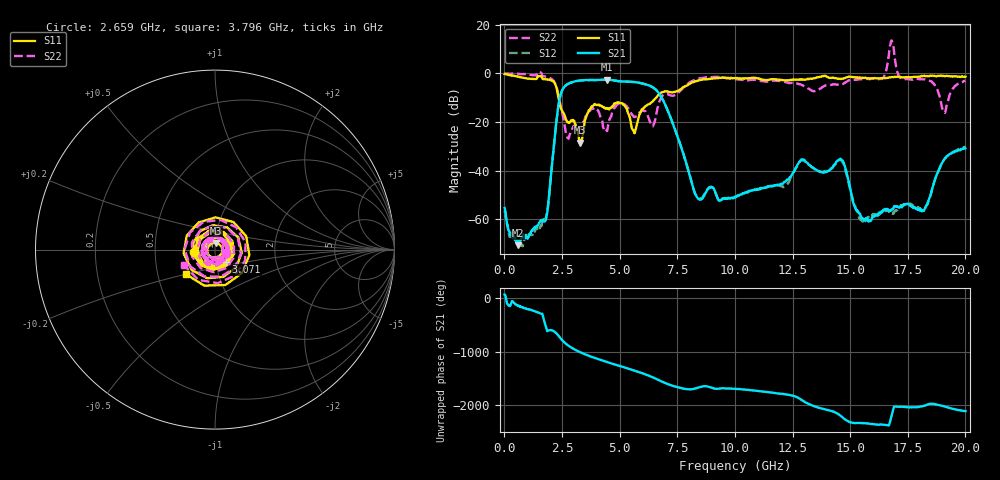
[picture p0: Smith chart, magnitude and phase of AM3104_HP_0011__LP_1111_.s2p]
!Created with skrf (http://scikit-rf.org).
# Hz S RI R 50.0
!freq ReS11 ImS11 ReS21 ImS21 ReS12 ImS12 ReS22 ImS22
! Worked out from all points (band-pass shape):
!   1601 points, 10 MHz to 20 GHz, reference 50 ohm
!   highest |S21| = -2.57 dB at 4.458 GHz (marker M1); lowest = -70.8 dB at 597.2 MHz (marker M2)
!   |S21| within 3 dB of the highest: 2.598 GHz to 6.423 GHz (3.825 GHz wide, 84.8 % of centre)
!   lowest |S11| = -28.5 dB at 3.283 GHz (marker M3), VSWR 1.08, Z = 50.3 + j3.76 ohm
!   |S11| at or under -10 dB: 2.347 GHz to 6.576 GHz (4.228 GHz wide, 94.8 % of centre)
!   |S22| runs from -26.8 to 13.6 dB; largest |S21 - S12| = 0.084
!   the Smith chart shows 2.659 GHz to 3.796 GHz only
!   S11 on the Smith chart (normalised r, x): 2.659 GHz: 0.79, -0.03; 3.071 GHz: 1.12, -0.15; 3.796 GHz: 0.70, -0.20
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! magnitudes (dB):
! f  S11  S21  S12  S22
! 10 MHz  -0.2  -55.4  -56.5  0.0
! 597.2 MHz  -1.3  -70.8  -69.4  -0.1
! 1.797 GHz  -2.4  -60.3  -59.6  -1.3
! 2.334 GHz  -9.3  -14.0  -14.0  -8.3
! 2.659 GHz  -18.6  -5.0  -4.9  -23.9
! 3.071 GHz  -20.8  -3.2  -3.2  -22.6
! 3.283 GHz  -28.5  -2.9  -3.0  -22.7
! 3.346 GHz  -27.3  -2.8  -2.9  -22.0
! 3.796 GHz  -13.5  -2.7  -2.7  -14.3
! 4.458 GHz  -14.3  -2.6  -2.6  -23.7
! 4.945 GHz  -11.8  -3.1  -3.2  -12.4
! 5.62 GHz  -24.1  -3.5  -3.5  -17.7
! 6.682 GHz  -8.8  -7.8  -7.8  -12.8
! 8.368 GHz  -3.0  -51.1  -50.8  -2.2
! 10.01 GHz  -2.0  -51.0  -50.8  -2.4
! 13.34 GHz  -2.2  -38.6  -38.6  -7.1
! 14.63 GHz  -2.2  -35.6  -36.0  -4.6
! 15.55 GHz  -1.8  -60.1  -60.8  -2.3
! 16.68 GHz  -1.7  -56.4  -57.0  7.3
! 18.2 GHz  -0.9  -56.5  -55.7  -2.4
! 19.06 GHz  -1.0  -35.6  -35.6  -15.7
! 20 GHz  -1.3  -30.8  -30.2  -3.0
